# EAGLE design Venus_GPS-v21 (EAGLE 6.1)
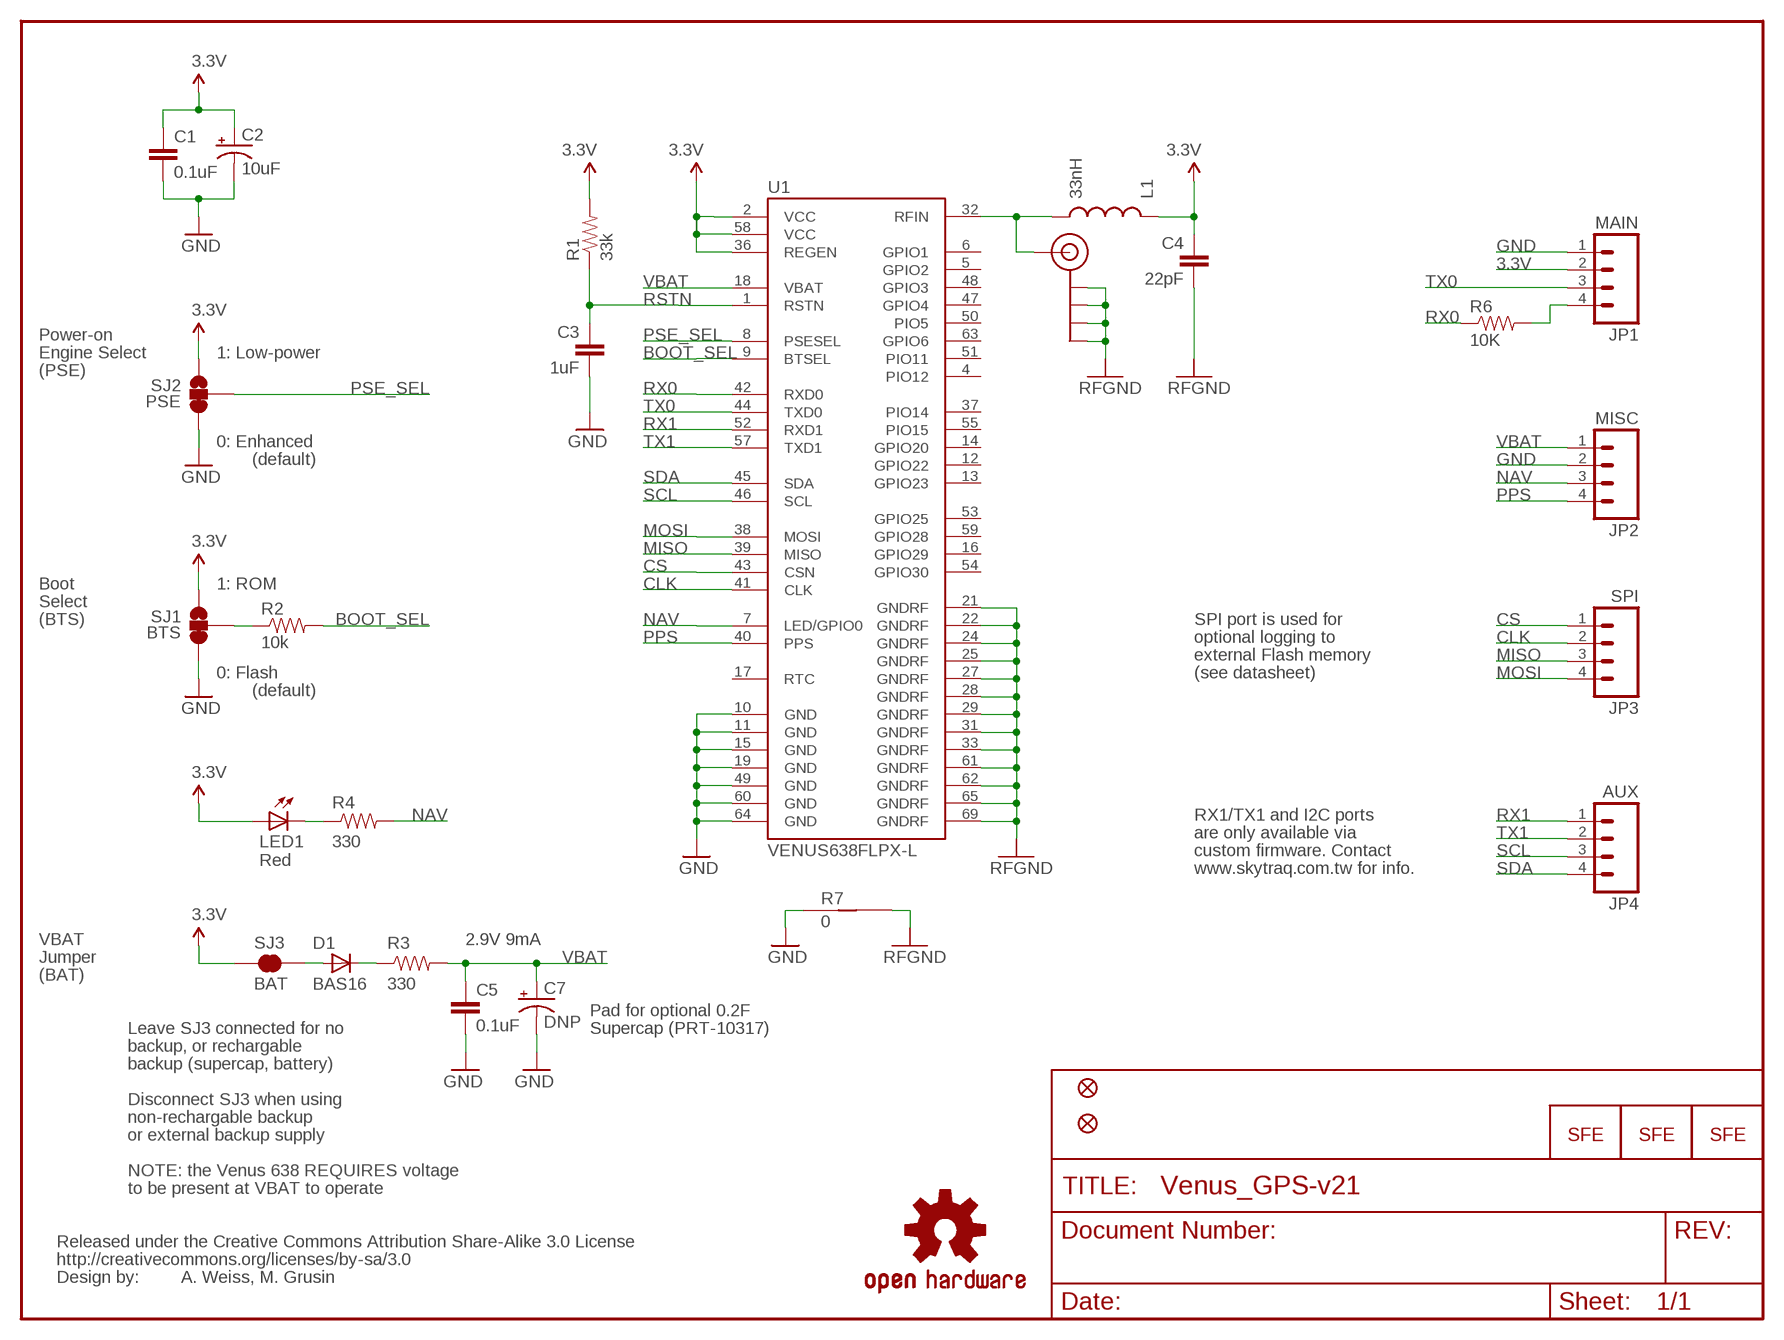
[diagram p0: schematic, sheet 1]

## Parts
C1  0.1uF  CAP0402-CAP  [0402-CAP]
C2  10uF  CAP_POL1206  [EIA3216]
C3  1uF  CAP0402-CAP  [0402-CAP]
C4  22pF  CAP0402-CAP  [0402-CAP]
C5  0.1uF  CAP0402-CAP  [0402-CAP]
C7  DNP  CAP_POLEN_J2  [EN_J2]
D1  BAS16  DIODESOD  [SOD-323]
JP1  MAIN  M04PTH  [1X04]
JP2  MISC  M04PTH  [1X04]
JP3  SPI  M04PTH  [1X04]
JP4  AUX  M04PTH  [1X04]
JP5  SMA_EDGE  [SMA-EDGE]
JP6  FIDUCIALUFIDUCIAL  [MICRO-FIDUCIAL]
JP7  FIDUCIALUFIDUCIAL  [MICRO-FIDUCIAL]
L1  33nH  INDUCTOR0402  [C0402]
LED1  Red  LED0603  [LED-0603]
LOGO1  LOGO-SFESK  [SFE-LOGO-FLAME]
LOGO2  LOGO-SFESK  [SFE-LOGO-FLAME]
LOGO3  LOGO-SFENW2  [SFE-NEW-WEB]
R1  33k  RESISTOR0402-RES  [0402-RES]
R2  10k  RESISTOR0402-RES  [0402-RES]
R3  330  RESISTOR0402-RES  [0402-RES]
R4  330  RESISTOR0402-RES  [0402-RES]
R6  10K  RESISTOR0402-RES  [0402-RES]
R7  0  GND-JUMP  [GND-JUMP]
SJ1  BTS  SOLDERJUMPER_2WAYPASTE2&3  [SJ_3_PASTE2&3]
SJ2  PSE  SOLDERJUMPER_2WAYPASTE2&3  [SJ_3_PASTE2&3]
SJ3  BAT  SOLDERJUMPERNC  [SJ_2S]
U1  VENUS638FLPX-L  [VENUS638FLPX]
U$4  OSHW-LOGOS  [OSHW-LOGO-S]
U$5  CREATIVE_COMMONS  [CREATIVE_COMMONS]

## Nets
3.3V: C1.1 C2.A(+) C4.1 JP1.2 L1.1 LED1.A R1.2 SJ1.1 SJ2.1 SJ3.1 U1.2(VCC) U1.36(REGEN) U1.58(VCC)
ANT: JP5.SIG(SIGNAL) L1.2 U1.32(RFIN)
BOOT_SEL: R2.2 U1.9(BTSEL)
CLK: JP3.2 U1.41(CLK)
CS: JP3.1 U1.43(CSN)
GND: C1.2 C2.C(-) C3.2 C5.2 C7.- JP1.1 JP2.2 R7.1 SJ1.3 SJ2.3 U1.10(GND) U1.11(GND) U1.15(GND) U1.19(GND) U1.49(GND) U1.60(GND) U1.64(GND)
MISO: JP3.3 U1.39(MISO)
MOSI: JP3.4 U1.38(MOSI)
N$1: LED1.C R4.1
N$2: R2.1 SJ1.2
N$3: D1.1(C) R3.1
N$6: D1.2(A) SJ3.2
NAV: JP2.3 R4.2 U1.7(LED/GPIO0)
PPS: JP2.4 U1.40(PPS)
PSE_SEL: SJ2.2 U1.8(PSESEL)
RFGND: C4.2 JP5.GND@0(GND) JP5.GND@1(GND) JP5.GND@2(GND) JP5.GND@3(GND) R7.2 U1.21(GNDRF) U1.22(GNDRF) U1.24(GNDRF) U1.25(GNDRF) U1.27(GNDRF) U1.28(GNDRF) U1.29(GNDRF) U1.31(GNDRF) U1.33(GNDRF) U1.61(GNDRF) U1.62(GNDRF) U1.65(GNDRF) U1.69(GNDRF)
RSTN: C3.1 R1.1 U1.1(RSTN)
RX0: R6.1 U1.42(RXD0)
RX1: JP4.1 U1.52(RXD1)
RX01: JP1.4 R6.2
SCL: JP4.3 U1.46(SCL)
SDA: JP4.4 U1.45(SDA)
TX0: JP1.3 U1.44(TXD0)
TX1: JP4.2 U1.57(TXD1)
VBAT: C5.1 C7.+ JP2.1 R3.2 U1.18(VBAT)
Unconnected: U1.4(PIO12) U1.5(GPIO2) U1.6(GPIO1) U1.12(GPIO22) U1.13(GPIO23) U1.14(GPIO20) U1.16(GPIO29) U1.17(RTC) U1.37(PIO14) U1.47(GPIO4) U1.48(GPIO3) U1.50(PIO5) U1.51(PIO11) U1.53(GPIO25) U1.54(GPIO30) U1.55(PIO15) U1.59(GPIO28) U1.63(GPIO6)

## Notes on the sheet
- Power-on
- Engine Select | 1: Low-power
- (PSE)
- RFGND | RFGND
- 0: Enhanced
- (default)
- Boot | 1: ROM
- Select
- (BTS) | SPI port is used for
- optional logging to
- external Flash memory
- 0: Flash | (see datasheet)
- (default)
- RX1/TX1 and I2C ports
- are only available via
- custom firmware. Contact
- RFGND | www.skytraq.com.tw for info.
- VBAT | 2.9V 9mA
- Jumper | RFGND
- (BAT)
- Pad for optional 0.2F
- Leave SJ3 connected for no | Supercap (PRT-10317)
- backup, or rechargable
- backup (supercap, battery)
- Disconnect SJ3 when using
- non-rechargable backup
- or external backup supply
- NOTE: the Venus 638 REQUIRES voltage
- to be present at VBAT to operate
- A. Weiss, M. Grusin

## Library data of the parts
C1 C3-C5 = SparkFun:CAP: Capacitor
C2 C7 = SparkFun:CAP_POL: Capacitor Polarized
D1 = SparkFun:DIODE: Diode
JP1-JP4 = SparkFun:M04: Header 4 Standard 4-pin 0.1" header. Use with straight break away headers (SKU : PRT-00116), right angle break away headers (PRT-00553), swiss pins (PRT-00743), machine pins (PRT-00117), and female headers (PRT-00115). Molex polarized connector foot print use with SKU : PRT-08231 with associated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
JP5 = SparkFun:SMA_EDGE: SMA Antenna Connector End launch SMA connector. The paste layer has been removed so that the connector can be hand soldered onto the board after reflow.
JP6 JP7 = SparkFun:FIDUCIAL: Fiducial Alignment Points
L1 = SparkFun:INDUCTOR: Inductors
LED1 = SparkFun:LED: LEDs
LOGO1-LOGO3 = SparkFun:LOGO-SFE: Spark Fun Electronics PCB Logo
R1-R4 R6 = SparkFun:RESISTOR: Resistor
R7 = mike-temp:GND-JUMP: Zero-Ohm trace for connecting different ground planes at a single point.
SJ1 SJ2 = SparkFun:SOLDERJUMPER_2WAY: Solder Jumper 2 way solder jumper
SJ3 = SparkFun:SOLDERJUMPER: Solder Jumper
U1 = mike-temp:VENUS638FLPX-L: Venus638FLPX-L GPS Receiver Venus638FLPx is a high performance, low cost, single chip GPS receiver targeting mobile consumer and cellular handset applications. It offers very low power consumption, high sensitivity, and best in class signal acquisition and time-to-first-fix performance.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
U$4 = SparkFun:OSHW-LOGO: Open Source Hardware Logo This logo indicates the piece of hardware it is found on incorporates a OSHW license and/or adheres to the definition of open source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
U$5 = SparkFun:CREATIVE_COMMONS

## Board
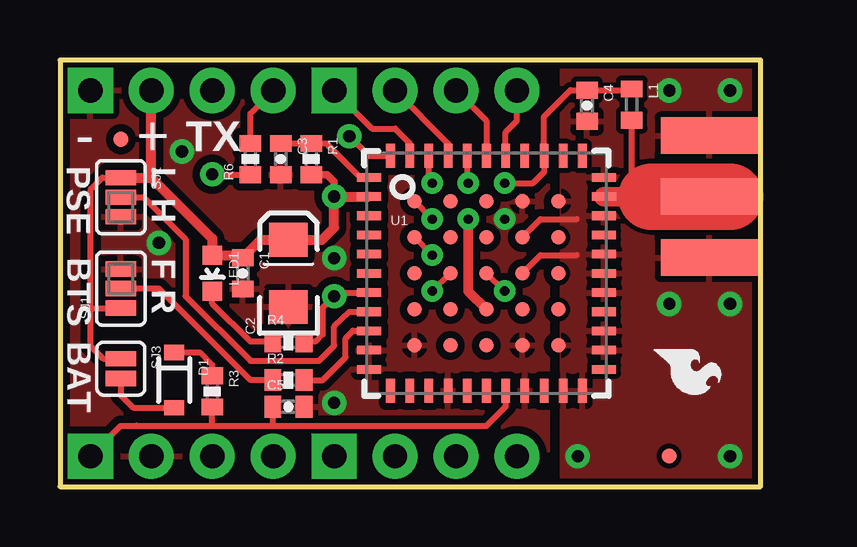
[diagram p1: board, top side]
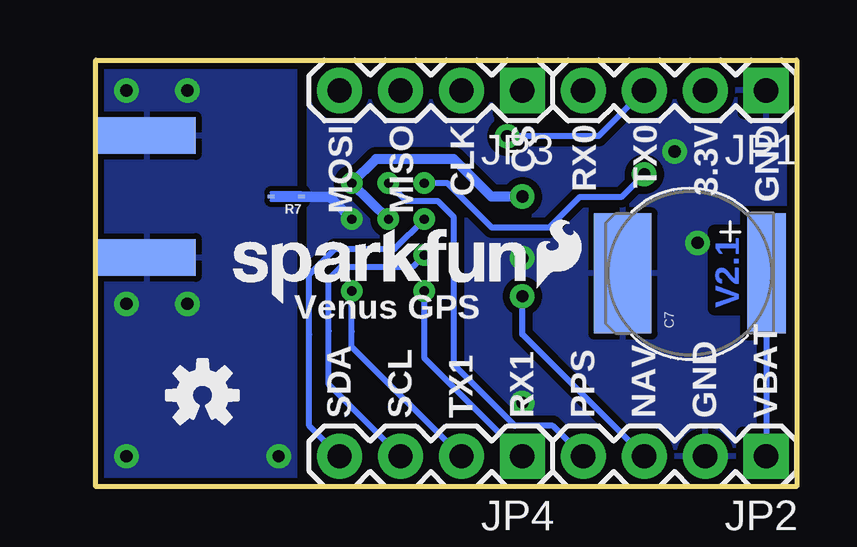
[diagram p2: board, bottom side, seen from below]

Size 29.21 x 17.78 mm. Coordinates in mm from the lower left corner, seen from the top.
Outline: 0,0 29.21,0 29.21,17.78 0,17.78 0,0
Copper layers (1*16): Top 0.035mm / dielectric 1.5mm / Bottom 0.035mm
Design rules: minimum track width 8mil, minimum drill 20mil, track to track 8mil, track to pad 8mil, pad to pad 8mil, via to via 8mil, smd to smd 8mil, copper to edge 10mil, drill to drill 8mil, minimum pad ring 12mil, minimum via ring 10mil, stop-mask expansion 4mil, vias tented up to drill 25mil, thermal gap 10mil

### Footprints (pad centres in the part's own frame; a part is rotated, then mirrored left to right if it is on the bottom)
0402-CAP = smd 0.7 x 0.9: 1 -0.65,0; 2 0.65,0
EIA3216 = smd 1.4 x 1.6: A 1.4,0; C -1.4,0
EN_J2 = smd 5 x 1.6: + 0,-3.2 | smd 5 x 2.4: - 0,2.8
SOD-323 = smd 0.63 x 0.83: 1 -1.15,0; 2 1.15,0
1X04 = drill 1.016 pad 1.88 square: 1 0,0 | drill 1.016 pad 1.88: 2 2.54,0; 3 5.08,0; 4 7.62,0
SMA-EDGE = smd 1.524 x 4.064: GND@0 0,0; GND@1 5.08,0; SIG 2.54,0 | smd 1.524 x 4.064 bottom: GND@2 0,0; GND@3 5.08,0
MICRO-FIDUCIAL = smd 0.635 x 0.635: 1 0,0
C0402 = smd 0.7 x 0.9: 1 -0.65,0; 2 0.65,0
LED-0603 = smd 0.8 x 0.8: A 0,-0.75; C 0,0.75
0402-RES = smd 0.7 x 0.9: 1 -0.65,0; 2 0.65,0
GND-JUMP = smd 0.305 x 0.152: 1 -0.635,0; 2 0.635,0
SJ_3_PASTE2&3 = smd 0.635 x 1.27: 1 -0.813,0; 2 0,0; 3 0.813,0
SJ_2S = smd 0.635 x 1.27: 1 -0.412,0; 2 0.412,0
VENUS638FLPX = smd 1 x 0.36: 1 -4.9,4; 2 -4.9,3.2; 3 -4.9,2.4; 4 -4.9,1.6; 5 -4.9,0.8; 6 -4.9,0; 7 -4.9,-0.8; 8 -4.9,-1.6; 9 -4.9,-2.4; 10 -4.9,-3.2; 11 -4.9,-4; 23 4.9,-4; 24 4.9,-3.2; 25 4.9,-2.4; 26 4.9,-1.6; 27 4.9,-0.8; 28 4.9,0; 29 4.9,0.8; 30 4.9,1.6; 31 4.9,2.4; 32 4.9,3.2; 33 4.9,4 | smd 0.36 x 1: 12 -4,-4.9; 13 -3.2,-4.9; 14 -2.4,-4.9; 15 -1.6,-4.9; 16 -0.8,-4.9; 17 0,-4.9; 18 0.8,-4.9; 19 1.6,-4.9; 20 2.4,-4.9; 21 3.2,-4.9; 22 4,-4.9; 34 4,4.9; 35 3.2,4.9; 36 2.4,4.9; 37 1.6,4.9; 38 0.8,4.9; 39 0,4.9; 40 -0.8,4.9; 41 -1.6,4.9; 42 -2.4,4.9; 43 -3.2,4.9; 44 -4,4.9 | smd 0.6 x 0.6: 45 -3,3; 46 -3,1.5; 47 -3,0; 48 -3,-1.5; 49 -3,-3; 50 -1.5,3; 51 -1.5,1.5; 52 -1.5,0; 53 -1.5,-1.5; 54 -1.5,-3; 55 0,3; 56 0,1.5; 57 0,0; 58 0,-1.5; 59 0,-3; 60 1.5,3; 61 1.5,1.5; 62 1.5,0; 63 1.5,-1.5; 64 1.5,-3; 65 3,3; 66 3,1.5; 67 3,0; 68 3,-1.5; 69 3,-3

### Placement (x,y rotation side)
C1  7.62,8.89 270 top
C2  9.53,8.89 90 top
C3  9.21,13.65 270 top
C4  21.97,15.88 270 top
C5  9.53,3.33 0 top
C7  4.45,8.89 90 bottom
D1  4.76,4.45 270 top
JP1  1.27,16.51 180 bottom
JP2  1.27,1.27 180 bottom
JP3  11.43,16.51 180 bottom
JP4  11.43,1.27 180 bottom
JP5  27.08,9.55 90 top
JP6  25.4,1.27 0 top
JP7  2.54,14.48 0 top
L1  23.84,15.93 270 top
LED1  6.35,8.89 180 top
LOGO1  24.77,5.71 270 top
LOGO2  10.83,8.29 0 bottom
LOGO3  23.5,7.62 0 bottom
R1  10.48,13.65 270 top
R2  9.53,4.45 0 top
R3  6.35,3.97 270 top
R4  9.53,6.05 0 top
R6  7.94,13.65 90 top
R7  21.27,12.09 180 bottom
SJ1  2.54,8.26 90 top
SJ2  2.54,12.06 270 top
SJ3  2.54,4.92 270 top
U1  17.78,8.89 0 top
U$4  24.77,3.81 0 bottom
U$5  not placed on the board

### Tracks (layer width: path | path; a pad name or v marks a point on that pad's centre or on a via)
3.3V  (via drill 0.38, 0.51)
  Top 0.254: SJ2.1 1.76,12.88 1.28,12.39 1.28,7.44 | U1.58 17.78,7.32 | v18.54,12.65 19.72,12.65 20.19,13.12 U1.36 20.18,15.42 20.32,15.56 21.29,16.52 C4.1 23.79,16.52 L1.1 | 1.28,7.44 SJ1.1 | 1.28,7.44 1.28,5.86 1.81,5.33 SJ3.1 | 7.52,9.64 C1.1
  Top 0.305: R1.2 11.13,13 11.43,12.7 v11.43,12.09
  Top 0.406: U1.58 17.02,8.15 v17.02,11.15 | SJ2.1 3.81,12.88 | 3.81,12.88 JP1.2 | U1.2 11.77,12.09 v11.43,12.09 11.43,10.79 10.93,10.29 C2.A 8.37,10.29 C1.1 | 7.52,9.64 LED1.A 6.35,10.34 3.81,12.88
  Bottom 0.406: v17.02,11.15 v18.54,12.65 17.54,13.65 14.29,13.65 12.72,12.09 v11.43,12.09
ANT
  Top 0.254: L1.2 23.84,12.38 24.13,12.09 | JP5.SIG
  Top 0.813: U1.32 24.13,12.09 24.66,12.09
  Top 2.769: 27.94,12.09 24.66,12.09 JP5.SIG
BOOT_SEL
  Top 0.254: U1.9 12.22,6.5 11.91,6.19 11.91,5.4 10.95,4.45 R2.2
CLK
  Top 0.254: U1.41 16.18,14.3 JP3.2
CS
  Top 0.254: U1.43 14.58,14.31 13.97,14.92 13.02,14.92 JP3.1
GND  (via drill 0.38, 0.51)
  Bottom 0.406: 19.48,12.09 U1.60 v18.54,11.15
  Bottom 0.445: R7.1 19.48,12.09
  other vias: 4.13,10.16 11.43,9.53 11.43,3.49 5.08,13.97
  pour Bottom (isolate 0.305): 0,17.78 20.32,17.78 20.32,0 0,0
  pour Top (isolate 0.305): 0,17.78 20.32,17.78 20.32,0 0,0
MISO
  Top 0.254: U1.39 17.78,15.24 JP3.3
MOSI
  Top 0.254: U1.38 18.58,14.77 19.05,15.24 JP3.4
N$1
  Top 0.254: R4.1 7.94,6.04 6.35,7.63 LED1.C
N$2
  Top 0.254: SJ1.2 4.13,8.26 7.94,4.45 R2.1
N$3
  Top 0.254: D1.1 5.83,5.59 6.35,5.08 R3.1
N$6
  Top 0.254: D1.2 3.06,3.29 2.54,3.81 SJ3.2
NAV  (via drill 0.51)
  Top 0.254: R4.2 10.65,6.04 10.95,6.35 10.95,7.14 10.95,7.46 v11.43,7.94 11.58,8.09 U1.7
  Bottom 0.254: JP2.3 11.43,6.35 v11.43,7.94
PPS  (via drill 0.38)
  Top 0.254: U1.40 16.99,12.7 v17.02,12.65
  Bottom 0.254: JP2.4 10.16,2.54 11.75,2.54 14.29,5.08 14.29,11.23 14.95,11.9 16.27,11.9 v17.02,12.65
PSE_SEL
  Top 0.254: 12.06,7.29 11.43,6.68 11.43,5.87 10.79,5.24 7.94,5.24 5.24,7.94 5.24,10.32 3.49,12.06 SJ2.2 | 12.06,7.29 U1.8 | 12.06,7.29
RFGND  (via drill 0.51)
  Top 0.254: U1.61 20.04,11.15 21.54,11.15 | U1.62 20.04,9.65 21.54,9.65
  other vias: 25.4,16.51 21.59,1.27 27.94,1.27 27.94,16.51 27.94,7.62 25.4,7.62
  pour Top: 20.95,17.78 20.95,0 29.21,0 29.21,17.78
  pour Bottom: 20.95,17.78 20.95,0 29.21,0 29.21,17.78
RSTN
  Top 0.254: C3.1 R1.1 11.1,14.3 12.51,12.89 U1.1
RX0  (via drill 0.38, 0.51)
  Top 0.254: U1.42 15.39,12.8 v15.52,12.65 | R6.1 6.37,13 v6.35,13.02
  Bottom 0.254: v15.52,12.65 14.55,12.65 12.7,10.79 10.32,10.79 9.05,12.06 7.3,12.06 v6.35,13.02
RX1  (via drill 0.38)
  Top 0.254: 16.2,8.89 U1.52 v15.52,8.15
  Bottom 0.254: v15.52,8.15 15.52,6.34 15.52,5.36 JP4.1
RX01
  Top 0.254: R6.2 7.94,15.56 JP1.4
SCL  (via drill 0.38)
  Top 0.254: v15.52,9.65 U1.46
  Bottom 0.254: JP4.3 19.51,4.27 19.51,6.49 19.51,8.64 18.99,9.18 16,9.18 v15.52,9.65
SDA  (via drill 0.38)
  Top 0.254: v15.52,11.15 U1.45
  Bottom 0.254: v15.52,11.15 16.76,9.91 19.25,9.91 20.32,8.84 20.32,6.35 20.32,2.54 JP4.4
TX0  (via drill 0.51)
  Top 0.254: U1.44 12.88,13.79 v12.06,14.61
  Bottom 0.254: v12.06,14.61 8.26,14.61 JP1.3
TX1  (via drill 0.38)
  Top 0.254: v18.54,8.15 U1.57
  Bottom 0.254: v18.54,8.15 18.54,6.48 18.54,5.84 JP4.2
VBAT
  Top 0.254: U1.18 18.59,3.35 17.78,2.54 8.89,2.54 | 3.17,2.54 2.54,2.54 JP2.1 | 3.17,2.54 6.35,2.54 | 6.35,2.54 8.89,2.54 | 6.35,2.54 R3.2 | 3.17,2.54 3.19,2.56 | C5.1 8.89,3.32 8.89,2.54
  Bottom 0.254: C7.+ 1.25,1.29 JP2.1

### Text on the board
Bottom: V2.1
tPlace: - | + | TX | PSE | L H | BTS | F R | BAT
bPlace: GND | 3.3V | TX0 | RX0 | CS | CLK | MISO | MOSI | Venus GPS | VBAT | GND | NAV | PPS | RX1 | TX1 | SCL | SDA
tValues: A. Weiss, M. Grusin
Document: 0.000" | 0.050" | 0.150" | 1.150" | 0.700" | 0.650" | 0.476" | 0.050" | 0.000" | 0.000"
